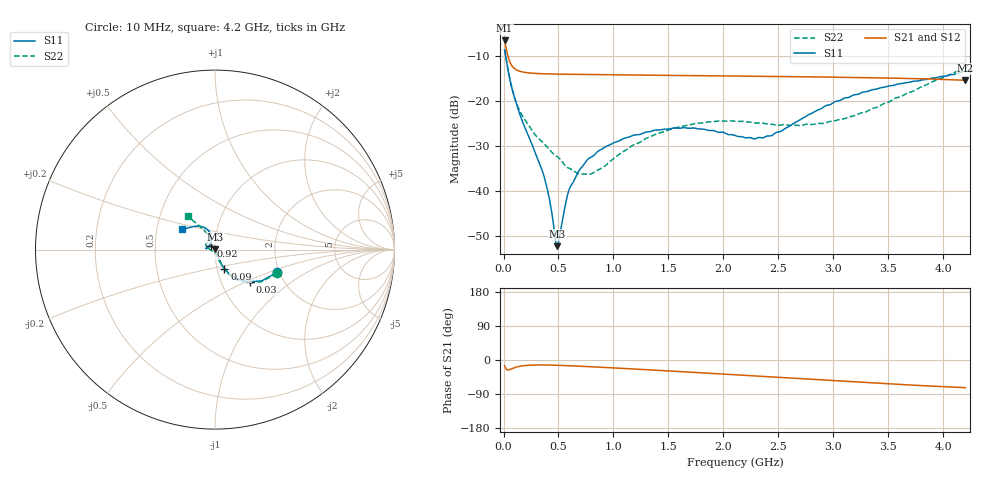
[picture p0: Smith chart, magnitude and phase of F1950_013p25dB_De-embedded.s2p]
! Integrated Device Technology
! Corporate Headquarters
! 6024 Silver Creek Valley Road
! San Jose, CA 95138  USA
! Phone:  1-408-284-8200
! Toll Free:  1-800-223-1366
! Webpage:  http://www.idt.com/
! Timing and RF Division
! 515 Groton Road, Suite 102
! Westford, MA 01886-6024
! Device:  F1950
! Description: 7-bit 0.25 dB Digital Step Attenuator
! Frequency:  150.0 -  4000.00 MHz
! Package:  4x4 mm Thin QFN Plastic Package: 24 pin
! Ports:  2 RF, 12 DC
!  Pin  1  = D0
!  Pin  2  = VDD
!  Pin  3  = Vmode
!  Pin  4  = GND
!  Pin  5  = RF1  =  Port 1
!  Pin  6  = GND
!  Pin  7  = GND
!  Pin  8  = GND
!  Pin  9  = GND
!  Pin 10  = GND
!  Pin 11  = GND
!  Pin 12  = GND
!  Pin 13  = GND
!  Pin 14  = RF2  =  Port 2
!  Pin 15  = GND
!  Pin 16  = LE
!  Pin 17  = CLK
!  Pin 18  = DATE
!  Pin 19  = D6
!  Pin 20  = D5
!  Pin 21  = D4
!  Pin 22  = D3
!  Pin 23  = D2
!  Pin 24  = D1
! State:  53
! Atten State:  13.25 dB
! Voltage:  +5.00 Volts
! Current:  Not Measured mA
! Data:  The device was measured on a the F195X evaluation board which has
!  individual transmission lines to the RF pins.  Data was collected
!  using a calibrated network analyzer.  The evaluation board was
!  de-embedded using a TRL calibration technique.
!  The reference plane is the edge of the package pin.
! Misc:  Board 2019
!  Action Tracker AT0250
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# GHz S dB R 50
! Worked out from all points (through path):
!   420 points, 10 MHz to 4.2 GHz, reference 50 ohm
!   highest |S21| = -6.60 dB at 10 MHz (marker M1); lowest = -15.4 dB at 4.2 GHz (marker M2)
!   group delay of S21, straight-line fit = 42.9 ps
!   lowest |S11| = -52.3 dB at 490 MHz (marker M3), VSWR 1.00, Z = 50.2 + j0.181 ohm
!   |S11| at or under -10 dB: 19.42 MHz to end of sweep
!   |S22| runs from -36.3 to -8.6 dB; largest |S21 - S12| = 0.00028
!   S11 on the Smith chart (normalised r, x): 10 MHz: 1.94, -0.57; 30 MHz: 1.36, -0.53; 90 MHz: 1.08, -0.24; 920 MHz: 0.95, +0.03; 4.2 GHz: 0.68, +0.16
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0.01  -8.68 -20.2  -6.60 -15.2  -6.60 -15.2  -8.61 -21.0
0.03  -11.56 -42.9  -9.04 -25.4  -9.04 -25.4  -11.48 -44.2
0.06  -15.57 -57.7  -11.50 -25.0  -11.49 -25.0  -15.32 -59.0
0.09  -18.47 -63.8  -12.62 -21.4  -12.62 -21.4  -18.38 -63.8
0.18  -25.11 -64.6  -13.63 -15.1  -13.63 -15.1  -23.65 -70.0
0.37  -36.88 -49.8  -14.01 -13.1  -14.01 -13.1  -29.56 -75.1
0.42  -42.11 -42.5  -14.04 -13.4  -14.04 -13.4  -30.90 -76.5
0.47  -50.51 -0.2  -14.07 -13.7  -14.07 -13.8  -32.11 -82.6
0.49  -52.29 48.1  -14.08 -13.9  -14.08 -13.9  -32.45 -84.4
0.51  -50.05 85.8  -14.09 -14.1  -14.09 -14.1  -32.84 -85.4
0.59  -40.24 119.9  -14.12 -15.0  -14.12 -15.0  -34.91 -97.0
0.71  -34.80 131.5  -14.16 -16.6  -14.16 -16.6  -36.26 -119.8
0.92  -30.34 143.9  -14.22 -19.6  -14.22 -19.7  -34.53 -163.1
1.17  -27.74 156.2  -14.29 -23.5  -14.29 -23.5  -29.96 174.2
1.41  -26.48 166.7  -14.34 -27.4  -14.34 -27.4  -27.19 164.9
1.73  -26.05 173.7  -14.42 -32.6  -14.41 -32.6  -25.11 156.2
2.11  -27.77 164.8  -14.51 -39.1  -14.50 -39.2  -24.56 146.4
2.43  -27.79 130.6  -14.59 -44.5  -14.58 -44.5  -25.18 135.6
2.81  -22.70 106.8  -14.69 -51.1  -14.68 -51.2  -25.26 119.4
3.19  -18.67 110.1  -14.82 -57.8  -14.81 -57.8  -23.31 113.5
3.51  -16.69 119.3  -14.95 -63.1  -14.95 -63.1  -20.21 116.3
4.2  -13.39 148.1  -15.45 -73.1  -15.44 -73.2  -12.43 129.3
